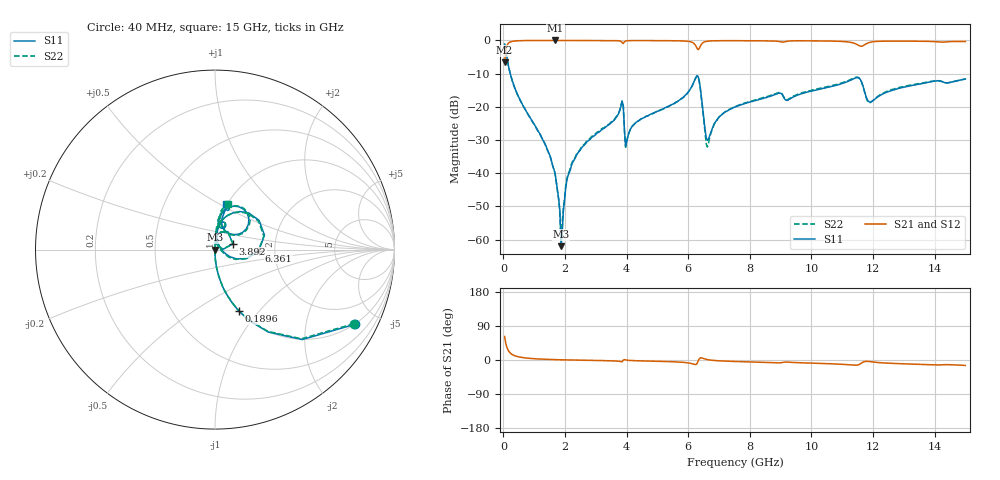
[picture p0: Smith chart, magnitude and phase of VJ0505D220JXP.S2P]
! VJ0505D220JXP
! MLCC placed on 25 mil thick microstrip substrate in series configuraton.
! DATE 06/29/2018  09:09
! CORRECTED  DATA
# GHz  S  MA  R  50.00
!  FREQ  S11M  S11A  S21M  S21A  S12M  S12A  S22M  S22A
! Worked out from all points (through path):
!   401 points, 40 MHz to 15 GHz, reference 50 ohm
!   highest |S21| = -0.01 dB at 1.686 GHz (marker M1); lowest = -6.6 dB at 40 MHz (marker M2)
!   group delay of S21, straight-line fit = 3.62 ps
!   lowest |S11| = -62.0 dB at 1.873 GHz (marker M3), VSWR 1.00, Z = 50 - j0.0791 ohm
!   |S11| at or under -10 dB: 223.7 MHz to end of sweep
!   |S22| runs from -60.3 to -1.1 dB; largest |S21 - S12| = 0.0026
!   S11 on the Smith chart (normalised r, x): 40 MHz: 0.99, -3.76; 189.6 MHz: 0.99, -0.79; 3.892 GHz: 1.22, +0.08; 6.361 GHz: 1.65, -0.02; 15 GHz: 0.99, +0.54
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0.04  0.8841 -28.1  0.4701 61.9  0.4703 62.0  0.8773 -28.1
0.1896  0.367 -68.9  0.9298 21.6  0.9306 21.5  0.3639 -68.8
0.601  0.1122 -84.2  0.9932 6.7  0.9936 6.7  0.1114 -84.2
1.3864  0.02537 -89.6  0.9982 1.9  0.999 1.9  0.02511 -90.9
1.6856  0.009485 -90.7  0.9989 1.0  0.9989 1.1  0.00939 -95.8
1.8726  0.0007968 -83.0  0.9971 0.6  0.9982 0.7  0.0009623 -154.0
1.9474  0.002657 88.7  0.9977 0.5  0.9979 0.5  0.00304 107.8
2.1344  0.01003 88.3  0.9977 0.1  0.9979 0.2  0.01057 93.2
2.5458  0.02438 88.2  0.9969 -0.5  0.9975 -0.5  0.02532 89.4
3.8174  0.1026 70.6  0.9673 -4.4  0.9679 -4.4  0.1041 71.6
3.8922  0.1052 17.6  0.8987 -0.6  0.899 -0.5  0.1043 18.2
4.0418  0.03601 77.3  0.991 -0.7  0.9915 -0.6  0.03561 82.2
5.0516  0.08779 85.2  0.9934 -3.4  0.9938 -3.4  0.08674 87.0
6.1736  0.2303 63.2  0.912 -10.9  0.9128 -10.9  0.2278 63.3
6.3606  0.2445 -1.3  0.7587 3.1  0.7592 3.1  0.239 -2.7
6.6224  0.03126 25.3  0.9732 1.1  0.9738 1.1  0.02481 30.7
7.52  0.09967 83.1  0.9908 -3.9  0.9915 -3.9  0.1012 87.0
10.0258  0.1738 82.0  0.985 -8.3  0.9862 -8.3  0.1787 83.2
11.4844  0.2751 56.6  0.8667 -13.5  0.8671 -13.4  0.2801 55.0
11.8958  0.1182 54.3  0.9354 -4.3  0.9357 -4.3  0.1151 56.2
12.5316  0.1716 77.1  0.9763 -8.5  0.9772 -8.5  0.1762 81.1
15  0.2619 76.2  0.9626 -14.3  0.9631 -14.3  0.2635 74.5
